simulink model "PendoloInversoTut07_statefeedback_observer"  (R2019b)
settings: Solver=ode4  StartTime=0  StopTime=10  FixedStep=0.0001  MaxStep=0.02  RelTol=1e-3  AbsTol=1e-6
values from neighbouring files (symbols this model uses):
  A = [0      1              0           0    [PendInvCarrello_Svolgimento.m]
  B = [ 0; (I+m*l^2)/p; 0; m*l/p]    [PendInvCarrello_Svolgimento.m]
  C = [1 0 0 0; 0 0 1 0]    [PendInvCarrello_Svolgimento.m]
  K = Kbar*inv(T)    [PendInvCarrello_Svolgimento.m]
  Lo = place(Ad',Cd',p_oss_des)'    [PendInvCarrello_Svolgimento.m]
  mu = dcgain(Gry)    [PendInvCarrello_Svolgimento.m]
  Tc = 0.02    [PendInvCarrello_Svolgimento.m]
  yzero = 0.2    [PendInvCarrello_Svolgimento.m]
undefined symbols (not defined in the file or in its folder): Ad, Bd, Cd, Reference

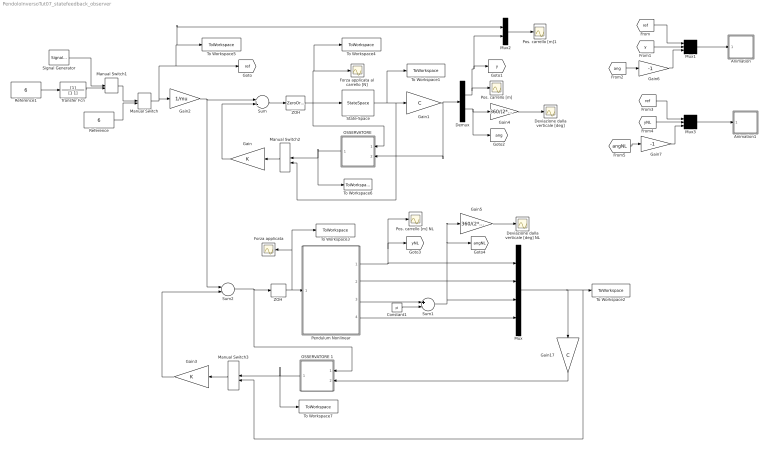
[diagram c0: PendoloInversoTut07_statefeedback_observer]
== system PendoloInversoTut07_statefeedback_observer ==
  Animation : Subsystem  mask(Pendulum plot){RefBlock=Reference}
      mask prompts: RefBlock "DC reference signal block name:"
      mask help: Pendulum plot
  Animation1 : Subsystem  mask(Pendulum plot){RefBlock=Reference}
      mask prompts: RefBlock "DC reference signal block name:"
      mask help: Pendulum plot
  Constant1 : Constant  Value=pi
  Demux : Demux  Outputs=2
  Deviazione dalla verticale [deg] NL : Scope
  Deviazione dalla verticale [deg] : Scope
  Forza applicata : Scope
  Forza applicata al carrello [N] : Scope
  Gain : Gain  Gain=K  Multiplication=Matrix(K*u)
  Gain1 : Gain  Gain=C  Multiplication=Matrix(K*u)
  Gain17 : Gain  Gain=C  Multiplication=Matrix(K*u)
  Gain2 : Gain  Gain=1/mu
  Gain3 : Gain  Gain=K  Multiplication=Matrix(K*u)
  Gain4 : Gain  Gain=360/(2*pi)
  Gain5 : Gain  Gain=360/(2*pi)
  Gain6 : Gain  Gain=-1
  Gain7 : Gain  Gain=-1
  Manual Switch : ManualSwitch  CurrentSetting=0
  Manual Switch1 : ManualSwitch
  Manual Switch2 : ManualSwitch
  Manual Switch3 : ManualSwitch
  Mux : Mux
  Mux1 : Mux  Inputs=3
  Mux2 : Mux  Inputs=2
  Mux3 : Mux  Inputs=3
  "OSSERVATORE " : Subsystem
  OSSERVATORE 1 : Subsystem
  Pendulum Nonlinear : Subsystem
  Pos. carrello [m] : Scope
  Pos. carrello [m] NL : Scope
  Pos. carrello [m]1 : Scope
  Reference : Constant  Value=6  VectorParams1D=off
  Reference1 : Constant  Value=6  VectorParams1D=off
  Signal Generator : SignalGenerator  Amplitude=6  Frequency=0.04  Units=rad/sec
  State-Space : StateSpace  A=A  B=B  C=eye(4)  D=zeros(4,1)  InitialCondition=[yzero ;0; 0; 0]
  Sum : Sum  Inputs=+-
  Sum1 : Sum  Inputs=+-
  Sum2 : Sum  Inputs=+-
  To Workspace1 : ToWorkspace  VariableName=x  SaveFormat=Timeseries  SampleTime=-1
  To Workspace2 : ToWorkspace  VariableName=x_NL  SaveFormat=Timeseries  SampleTime=-1
  To Workspace3 : ToWorkspace  VariableName=F_NL  SaveFormat=Timeseries  SampleTime=-1
  To Workspace4 : ToWorkspace  VariableName=F  SaveFormat=Timeseries  SampleTime=-1
  To Workspace5 : ToWorkspace  VariableName=Ref  SaveFormat=Timeseries  SampleTime=-1
  To Workspace6 : ToWorkspace  VariableName=xhat  SaveFormat=Timeseries  SampleTime=-1
  To Workspace7 : ToWorkspace  VariableName=xhatNL  SaveFormat=Timeseries  SampleTime=-1
  Transfer Fcn : TransferFcn  Denominator=[1 1]
  ZOH : ZeroOrderHold  SampleTime=Tc
  "ZOH " : ZeroOrderHold  SampleTime=Tc
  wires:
  Mux1/1 -> Animation/1(in_1)
  Sum/1 -> ZOH/1
  Demux/1 -> Mux2/2, [y], Pos. carrello [m]/1
  State-Space/1 -> Manual Switch2/2, Gain1/1, To Workspace1/1
  Demux/2 -> [ang], Gain4/1
  Gain2/1 -> Sum2/1, Sum/1
  [y] -> Mux1/2
  Constant1/1 -> Sum1/2
  Pendulum Nonlinear/1(CarrPos) -> [yNL], Pos. carrello [m] NL/1, Mux/1
  Pendulum Nonlinear/2(CarrVel) -> Mux/2
  Pendulum Nonlinear/3(Angle) -> Sum1/1
  Sum1/1 -> Mux/3, Gain5/1, [angNL]
  Pendulum Nonlinear/4(AngleDer) -> Mux/4
  Mux/1 -> Manual Switch3/2, To Workspace2/1, Gain17/1
  Gain3/1 -> Sum2/2
  "ZOH "/1 -> Forza applicata/1, To Workspace3/1, Pendulum Nonlinear/1(F)
  Manual Switch/1 -> Mux2/1, To Workspace5/1, [ref], Gain2/1
  Reference/1 -> Manual Switch/2
  [ref] -> Mux1/1
  Gain4/1 -> Deviazione dalla verticale [deg]/1
  Gain5/1 -> Deviazione dalla verticale [deg] NL/1
  Reference1/1 -> Transfer Fcn/1
  Transfer Fcn/1 -> Manual Switch1/2
  Signal Generator/1 -> Manual Switch1/1
  Manual Switch1/1 -> Manual Switch/1
  Mux2/1 -> Pos. carrello [m]1/1
  [ref] -> Mux3/1
  Mux3/1 -> Animation1/1(in_1)
  [yNL] -> Mux3/2
  Gain6/1 -> Mux1/3
  [ang] -> Gain6/1
  [angNL] -> Gain7/1
  Gain7/1 -> Mux3/3
  Sum2/1 -> OSSERVATORE 1/1(u(k)), "ZOH "/1
  ZOH/1 -> "OSSERVATORE "/1(u(k)), To Workspace4/1, Forza applicata al carrello [N]/1, State-Space/1
  Gain1/1 -> Demux/1, "OSSERVATORE "/2(y(k))
  "OSSERVATORE "/1(x hat) -> Manual Switch2/1, To Workspace6/1
  Gain/1 -> Sum/2
  Gain17/1 -> OSSERVATORE 1/2(y(k))
  OSSERVATORE 1/1(x hat) -> Manual Switch3/1, To Workspace7/1
  Manual Switch2/1 -> Gain/1
  Manual Switch3/1 -> Gain3/1

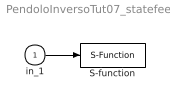
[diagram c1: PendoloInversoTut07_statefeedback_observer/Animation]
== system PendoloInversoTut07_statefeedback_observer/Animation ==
  in_1 : Inport
  S-function : S-Function  FunctionName=pendan_file  Parameters=RefBlock  SFunctionDeploymentMode=off  EnableBusSupport=off
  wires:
  in_1/1 -> S-function/1

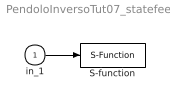
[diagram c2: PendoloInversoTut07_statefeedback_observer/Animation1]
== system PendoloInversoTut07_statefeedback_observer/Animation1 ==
  in_1 : Inport
  S-function : S-Function  FunctionName=pendan_fileNL  Parameters=RefBlock  SFunctionDeploymentMode=off  EnableBusSupport=off
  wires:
  in_1/1 -> S-function/1

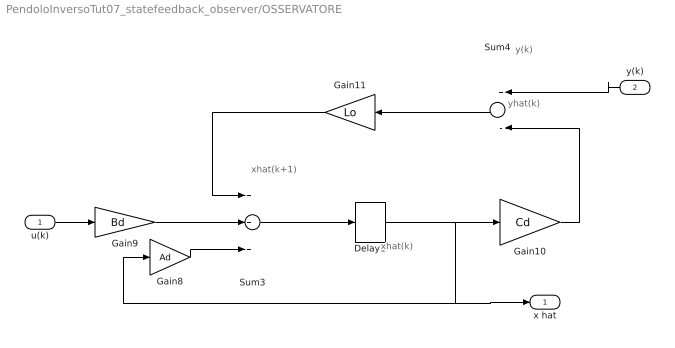
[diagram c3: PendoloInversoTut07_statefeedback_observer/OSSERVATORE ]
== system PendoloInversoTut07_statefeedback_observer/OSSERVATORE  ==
  note: xhat(k)
  note: yhat(k)
  note: y(k)
  note: xhat(k+1)
  u(k) : Inport
  y(k) : Inport  Port=2
  Delay1 : Delay  DelayLength=1  InitialCondition=0  SampleTime=Tc
  Gain10 : Gain  Gain=Cd  Multiplication=Matrix(K*u)
  Gain11 : Gain  Gain=Lo  Multiplication=Matrix(K*u)
  Gain8 : Gain  Gain=Ad  Multiplication=Matrix(K*u)
  Gain9 : Gain  Gain=Bd  Multiplication=Matrix(K*u)
  Sum3 : Sum  Inputs=+++
  Sum4 : Sum  Inputs=+-
  x hat : Outport
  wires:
  Sum4/1 -> Gain11/1
  Gain10/1 -> Sum4/2
  Gain8/1 -> Sum3/3
  y(k)/1 -> Sum4/1
  Gain9/1 -> Sum3/2
  Gain11/1 -> Sum3/1
  Sum3/1 -> Delay1/1
  Delay1/1 -> x hat/1, Gain8/1, Gain10/1
  u(k)/1 -> Gain9/1

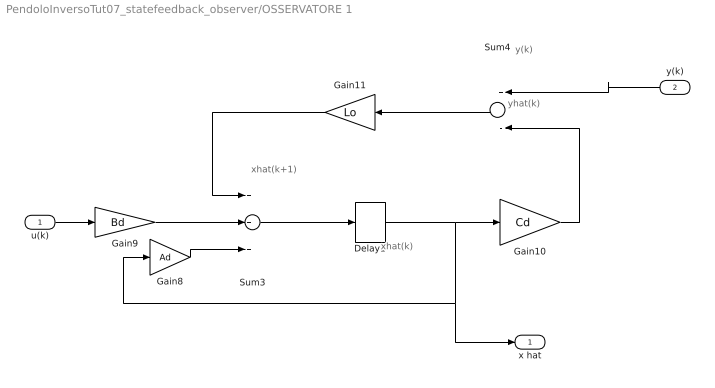
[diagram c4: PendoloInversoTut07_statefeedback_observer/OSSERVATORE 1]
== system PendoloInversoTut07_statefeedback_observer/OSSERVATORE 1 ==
  note: xhat(k+1)
  note: y(k)
  note: yhat(k)
  note: xhat(k)
  u(k) : Inport
  y(k) : Inport  Port=2
  Delay1 : Delay  DelayLength=1  InitialCondition=0  SampleTime=Tc
  Gain10 : Gain  Gain=Cd  Multiplication=Matrix(K*u)
  Gain11 : Gain  Gain=Lo  Multiplication=Matrix(K*u)
  Gain8 : Gain  Gain=Ad  Multiplication=Matrix(K*u)
  Gain9 : Gain  Gain=Bd  Multiplication=Matrix(K*u)
  Sum3 : Sum  Inputs=+++
  Sum4 : Sum  Inputs=+-
  x hat : Outport
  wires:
  u(k)/1 -> Gain9/1
  Delay1/1 -> Gain10/1, Gain8/1, x hat/1
  Sum3/1 -> Delay1/1
  Gain11/1 -> Sum3/1
  Gain9/1 -> Sum3/2
  y(k)/1 -> Sum4/1
  Gain8/1 -> Sum3/3
  Gain10/1 -> Sum4/2
  Sum4/1 -> Gain11/1

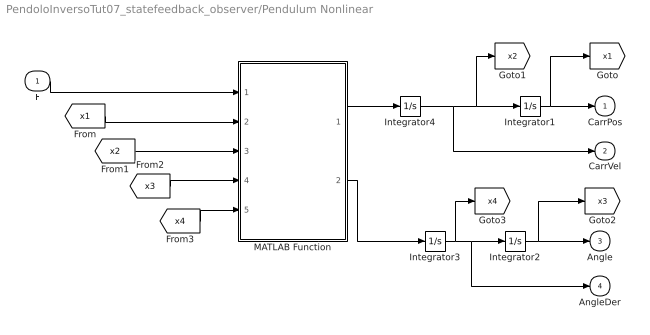
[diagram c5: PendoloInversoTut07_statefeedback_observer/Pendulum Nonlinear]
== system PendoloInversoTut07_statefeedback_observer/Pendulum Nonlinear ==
  F : Inport
  Integrator1 : Integrator  InitialCondition=yzero
  Integrator2 : Integrator  InitialCondition=pi
  Integrator3 : Integrator
  Integrator4 : Integrator
  MATLAB Function : MATLAB Function  TreatAsAtomicUnit=on
  CarrPos : Outport  InitialOutput=0  VectorParamsAs1DForOutWhenUnconnected=off
  CarrVel : Outport  Port=2  InitialOutput=0  VectorParamsAs1DForOutWhenUnconnected=off
  Angle : Outport  Port=3  InitialOutput=0  VectorParamsAs1DForOutWhenUnconnected=off
  AngleDer : Outport  Port=4  InitialOutput=0  VectorParamsAs1DForOutWhenUnconnected=off
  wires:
  Integrator1/1 -> [x1], CarrPos/1
  MATLAB Function/2(teta_ddot) -> Integrator3/1
  MATLAB Function/1(yddot) -> Integrator4/1
  Integrator4/1 -> CarrVel/1, [x2], Integrator1/1
  F/1 -> MATLAB Function/1(F)
  Integrator3/1 -> [x4], AngleDer/1, Integrator2/1
  Integrator2/1 -> [x3], Angle/1
  [x1] -> MATLAB Function/2(x1)
  [x2] -> MATLAB Function/3(x2)
  [x3] -> MATLAB Function/4(x3)
  [x4] -> MATLAB Function/5(x4)

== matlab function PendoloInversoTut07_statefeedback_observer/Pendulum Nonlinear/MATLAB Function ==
function [yddot,teta_ddot] = fcn(F,x1,x2,x3,x4)

M = 0.5;
m = 0.2;
b = 0.1;
I = 0.006;
l = 0.3;
g = 9.8;

Delta=(M+m)*(I+m*l^2)-m^2*l^2*cos(x3)^2;

yddot = -b*(I+m*l^2)*x2/Delta+m*l*x4^2*sin(x3)/Delta+m^2*g*l^2*sin(x3)*cos(x3)/Delta+(I+m*l^2)*F/Delta;

teta_ddot=m*l*b*cos(x3)*x2/Delta-m^2*l^2*x4^2*sin(x3)*cos(x3)/Delta-(M+m)*m*g*l*sin(x3)/Delta-m*l*cos(x3)*F/Delta;
